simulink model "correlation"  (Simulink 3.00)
settings: Solver=ode45  StartTime=0.0  StopTime=10  RelTol=1e-3

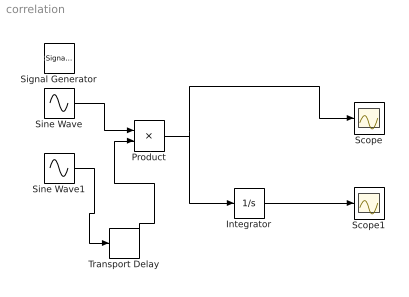
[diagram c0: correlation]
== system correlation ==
  Integrator : Integrator  ExternalReset=none  InitialConditionSource=internal  InitialCondition=0  LimitOutput=off  UpperSaturationLimit=inf  LowerSaturationLimit=-inf  ShowSaturationPort=off  ShowStatePort=off  AbsoluteTolerance=auto
  Product : Product  Inputs=2  SaturateOnIntegerOverflow=on
  Scope : Scope
  Scope1 : Scope
  Signal Generator : SignalGenerator  WaveForm=square  Amplitude=1  Frequency=1  Units=Hertz
  Sine Wave : Sin  Amplitude=1  Frequency=1  Phase=0  SampleTime=0
  Sine Wave1 : Sin  Amplitude=1  Frequency=0.5  Phase=0  SampleTime=0
  Transport Delay : TransportDelay  DelayTime=0.5  InitialInput=0  BufferSize=1024
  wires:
  Product/1 -> Scope/1, Integrator/1
  Integrator/1 -> Scope1/1
  Sine Wave/1 -> Product/1
  Transport Delay/1 -> Product/2
  Sine Wave1/1 -> Transport Delay/1
